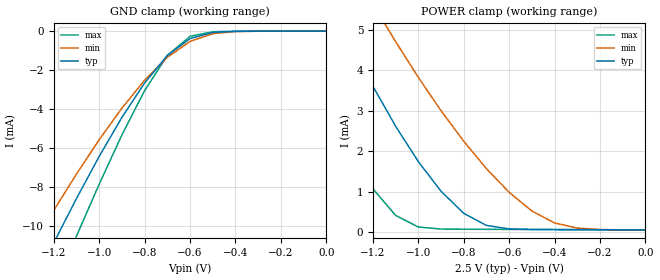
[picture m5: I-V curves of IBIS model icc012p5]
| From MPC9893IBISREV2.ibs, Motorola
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|This model is an Input with a 25,000 ohm Pull_down at 3.3V
[Model]   icc012p5
Model_type   Input
Polarity   Non-Inverting
Vmeas=1.25
Vinl=.7
Vinh=1.7
| Variable   typ   min   max
C_comp   5p   5p   5p
[Temperature Range]   27.00   100.00   -45.00
[Power Clamp Reference]   2.50V   2.25V   2.75V
[Gnd Clamp Reference]   0.000V   0.000V   0.000V
[Voltage Range]   2.50V   2.25V   2.75V
[Pulldown Reference]   0.000V   0.000V   0.000V
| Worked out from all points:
|   GND clamp passes 1 mA (typ) near -0.67 V on its own axis
|   POWER clamp passes 1 mA (typ) near -0.90 V on its own axis
[GND_clamp]
|   voltage   I(typ)   I(mim)   I(max)
-2.5V     -43.45mA   -37.55mA   -49.95mA
-1.3V     -13.19mA   -11.13mA   -16.03mA
-1.2V     -10.84mA   -9.179mA   -13.24mA
-1.1V     -8.57mA    -7.315mA   -10.5mA
-1V       -6.414mA   -5.56mA    -7.834mA
-900mV    -4.418mA   -3.945mA   -5.315mA
-800mV    -2.655mA   -2.515mA   -3.045mA
-700mV    -1.251mA   -1.342mA   -1.246mA
-600mV    -381.4uA   -529.5uA   -268.1uA
-500mV    -68.55uA   -130uA     -34.68uA
-400mV    -13.34uA   -24.07uA   -9.13uA
1.08fV    -5.997pA   -194.8pA   -2.759pA
[POWER_clamp]
|   voltage   I(typ)   I(min)   I(max)
-2.5V     21.34mA    20.61mA    21.17mA
-1.6V     8.368mA    9.807mA    5.933mA
-1.5V     7.082mA    8.714mA    4.497mA
-1.3V     4.687mA    6.629mA    2.018mA
-1.2V     3.603mA    5.646mA    1.064mA
-1.1V     2.613mA    4.709mA    405.6uA
-1V       1.738mA    3.824mA    120.9uA
-800mV    458.6uA    2.242mA    65.81uA
-700mV    160.2uA    1.563mA    63.68uA
-500mV    60.74uA    516.4uA    59.7uA
-400mV    57.78uA    221.5uA    57.71uA
1.08fV    49.75uA    49.79uA    49.75uA
